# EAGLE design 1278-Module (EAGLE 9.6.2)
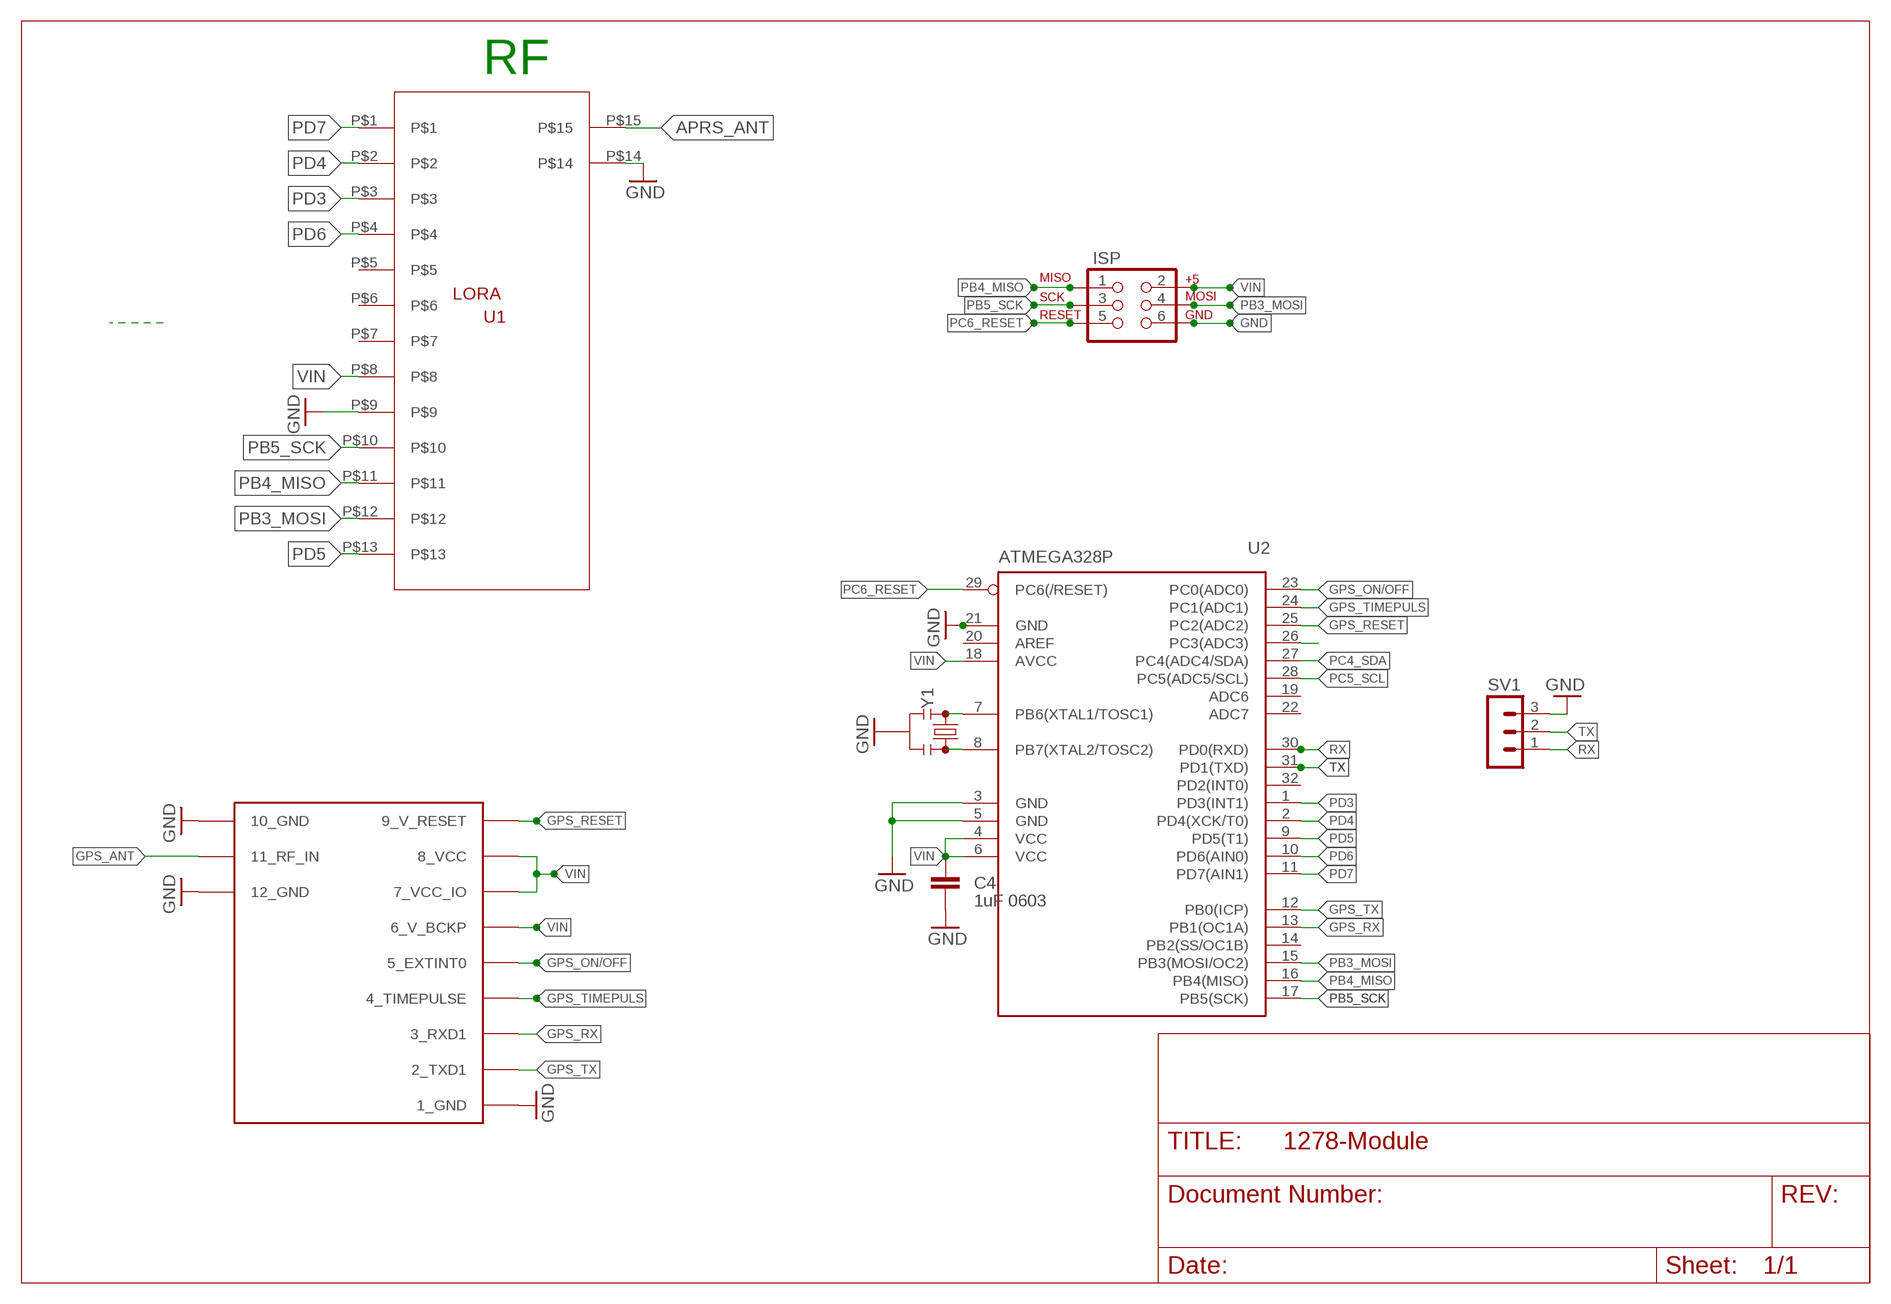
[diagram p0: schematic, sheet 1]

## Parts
C4  1uF 0603  C-EUC0603K  [C0603K]
ISP  AVR_SPI_PRG_6PTH  [2X3]
SV1  MA03-1  [MA03-1]
U1  LORA  [LORA_DRF]
U2  ATMEGA328P  MEGA8-AI  [TQFP32-08]
U$2  UBLOX_MAX  [UBLOX_MAX]
Y1  RESONATORSMD-4.5X2.0  [RESONATOR-SMD-4.5X2.0]

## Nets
APRS_ANT: U1.P$15
GND: C4.2 ISP.6 SV1.3 U1.P$9 U1.P$14 U2.3(GND) U2.5(GND) U2.21(GND) U$2.1_GND U$2.10_GND U$2.12_GND Y1.2
GPS_ANT: U$2.11_RF_IN
GPS_ON/OFF: U2.23(PC0(ADC0)) U$2.5_EXTINT0
GPS_RESET: U2.25(PC2(ADC2)) U$2.9_V_RESET
GPS_RX: U2.13(PB1(OC1A)) U$2.3_RXD1
GPS_TIMEPULS: U2.24(PC1(ADC1)) U$2.4_TIMEPULSE
GPS_TX: U2.12(PB0(ICP)) U$2.2_TXD1
N$1: U2.8(PB7(XTAL2/TOSC2)) Y1.3
N$2: U2.7(PB6(XTAL1/TOSC1)) Y1.1
N$10: U2.26(PC3(ADC3))
PB3_MOSI: ISP.4 U1.P$12 U2.15(PB3(MOSI/OC2))
PB4_MISO: ISP.1 U1.P$11 U2.16(PB4(MISO))
PB5_SCK: ISP.3 U1.P$10 U2.17(PB5(SCK))
PC4_SDA: U2.27(PC4(ADC4/SDA))
PC5_SCL: U2.28(PC5(ADC5/SCL))
PC6_RESET: ISP.5 U2.29(PC6(/RESET))
PD3: U1.P$3 U2.1(PD3(INT1))
PD4: U1.P$2 U2.2(PD4(XCK/T0))
PD5: U1.P$13 U2.9(PD5(T1))
PD6: U1.P$4 U2.10(PD6(AIN0))
PD7: U1.P$1 U2.11(PD7(AIN1))
RX: SV1.1 U2.30(PD0(RXD))
TX: SV1.2 U2.31(PD1(TXD))
VIN: C4.1 ISP.2 U1.P$8 U2.4(VCC) U2.6(VCC) U2.18(AVCC) U$2.6_V_BCKP U$2.7_VCC_IO U$2.8_VCC
Unconnected: U1.P$5 U1.P$6 U1.P$7 U2.14(PB2(SS/OC1B)) U2.19(ADC6) U2.20(AREF) U2.22(ADC7) U2.32(PD2(INT0))

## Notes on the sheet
- RF

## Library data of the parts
C4 = rcl:C-EU: CAPACITOR, European symbol; SPICEPREFIX: C
ISP = SparkFun:AVR_SPI_PRG_6: AVR ISP 6 Pin This is the reduced ISP connector for AVR programming. Common on Arduino. This footprint will take up less PCB space and can be used with a 10-pin to 6-pin adapter such as SKU: BOB-08508
SV1 = con-lstb:MA03-1: PIN HEADER; OC_FARNELL: unknown; OC_NEWARK: unknown
U1 = lora:LORA
U2 = atmel:MEGA8: MICROCONTROLLER 8 Kbytes FLASH, 1 kbytes SRAM, 512 bytes EEPROM, USART, 6-channel 10 bit ADC, 2-channel 8 bit ADC Pin compatible with Atmega48, ATMega88, ATMega168 Source: avr.lbr; MPN: ATMEGA8-16AU; OC_FARNELL: 9171371; OC_NEWARK: 73M8863
U$2 = Max gps:UBLOX_MAX: UBLOX MAX
Y1 = SparkFun-Clocks:RESONATOR: Resonators (Generic) Ceramic resonators are clock-generating components, often used to control timing in microcontrollers. They usually have 3 pins: two pins for oscillation, and one pin for ground. Compared to crystals, resonators have worse tolerance, but are usually much cheaper. Plus, they have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

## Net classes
0 default: width 0.152 mm, drill 0.305 mm, clearance 0.152 mm
1 vcc: width 0.152 mm, clearance 0.152 mm

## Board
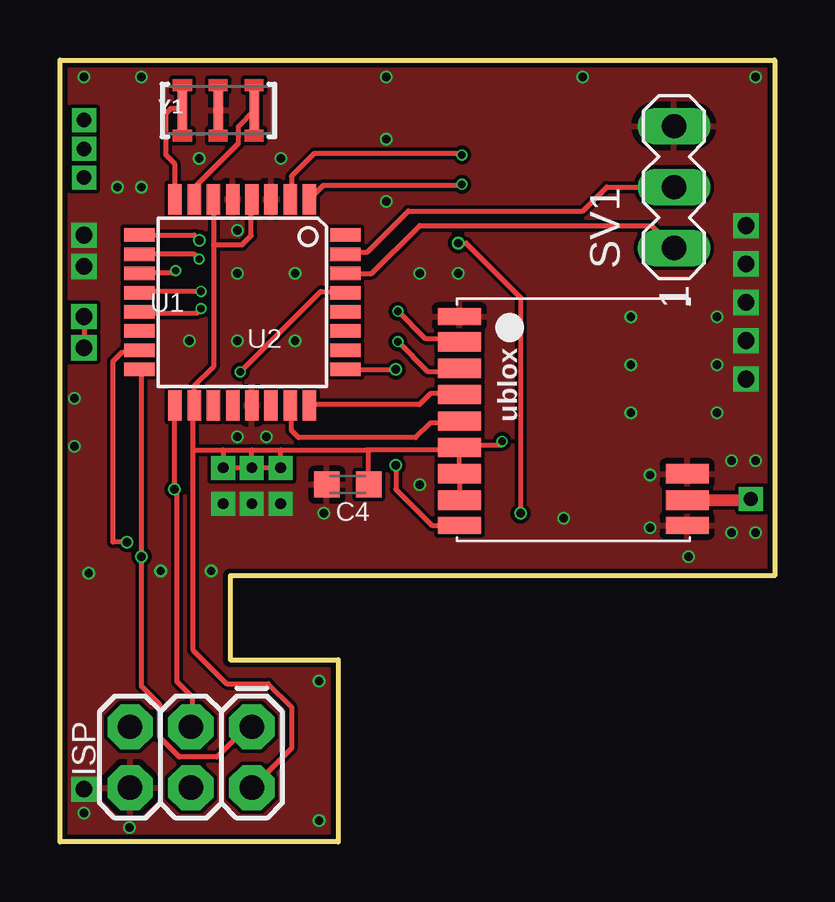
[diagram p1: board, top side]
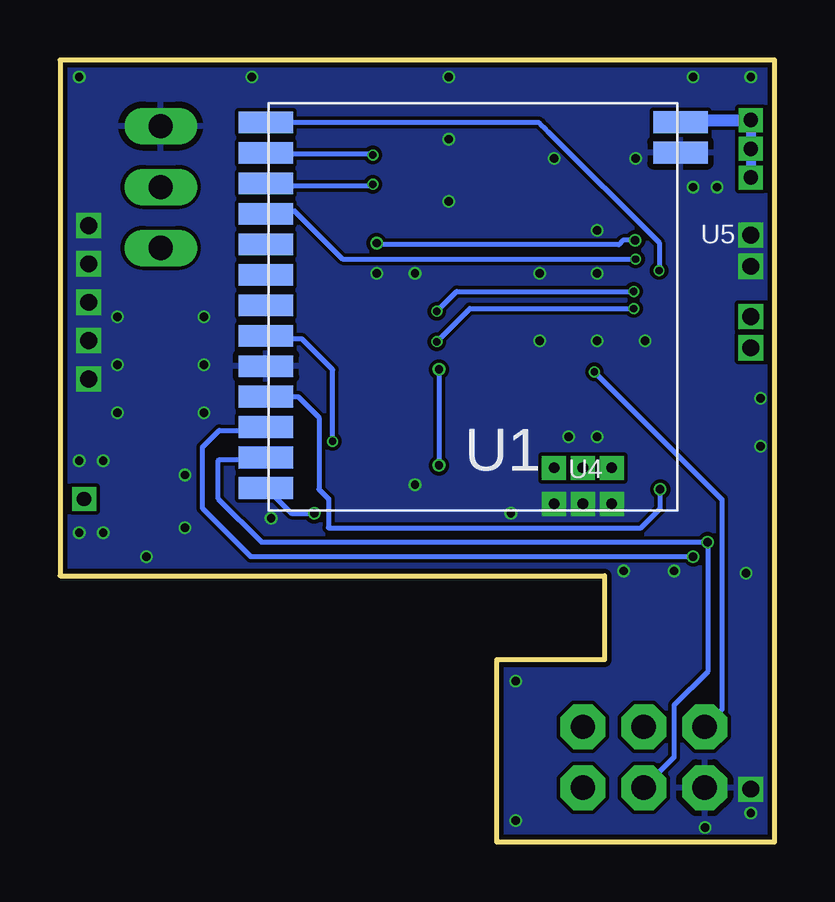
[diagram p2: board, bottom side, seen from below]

Size 29.8 x 32.6 mm. Coordinates in mm from the lower left corner, seen from the top.
Outline: 0,32.6 29.8,32.6 29.8,11.1 7.1,11.1 7.1,7.6 11.6,7.6 11.6,0 0,0 0,32.6
Copper layers (1*16): Top 0.035559375mm / dielectric 1.6mm / Bottom 0.035559375mm
Design rules "jlcpcb2layer *": minimum track width 5mil, minimum drill 12mil, track to track 5mil, track to pad 5mil, pad to pad 5mil, via to via 5mil, smd to smd 5mil, copper to edge 8mil, drill to drill 6mil, minimum pad ring 5mil, minimum via ring 3mil, stop-mask expansion 2.5mil, vias tented up to drill 14mil, thermal gap 10mil

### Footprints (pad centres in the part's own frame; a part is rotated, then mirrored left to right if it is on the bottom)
C0603K = smd 1.05 x 1.08: 1 -0.875,0; 2 0.875,0
2X3 = drill 1.016 pad 1.88 octagon: 1 0,0; 2 0,2.54; 3 2.54,0; 4 2.54,2.54; 5 5.08,0; 6 5.08,2.54
MA03-1 = drill 1.016 long: 1 -2.54,0; 2 0,0; 3 2.54,0
LORA_DRF = smd 2.27 x 0.9: P$1 -8.609,7.497; P$2 -8.609,6.227; P$3 -8.608,4.958; P$4 -8.608,3.688; P$5 -8.609,2.417; P$6 -8.609,1.147; P$7 -8.608,-0.122; P$8 -8.608,-1.392; P$9 -8.61,-2.663; P$10 -8.61,-3.933; P$11 -8.609,-5.202; P$12 -8.609,-6.472; P$13 -8.609,-7.743; P$14 8.673,6.235; P$15 8.675,7.506
TQFP32-08 = smd 1.27 x 0.559: 1 -4.293,2.8; 2 -4.293,2; 3 -4.293,1.2; 4 -4.293,0.4; 5 -4.293,-0.4; 6 -4.293,-1.2; 7 -4.293,-2; 8 -4.293,-2.8; 17 4.293,-2.8; 18 4.293,-2; 19 4.293,-1.2; 20 4.293,-0.4; 21 4.293,0.4; 22 4.293,1.2; 23 4.293,2; 24 4.293,2.8 | smd 0.559 x 1.27: 9 -2.8,-4.293; 10 -2,-4.293; 11 -1.2,-4.293; 12 -0.4,-4.293; 13 0.4,-4.293; 14 1.2,-4.293; 15 2,-4.293; 16 2.8,-4.293; 25 2.8,4.293; 26 2,4.293; 27 1.2,4.293; 28 0.4,4.293; 29 -0.4,4.293; 30 -1.2,4.293; 31 -2,4.293; 32 -2.8,4.293
UBLOX_MAX = smd 1.8 x 0.7: 1_GND 4.95,-4.4; 9_V_RESET 4.95,4.3; 10_GND -4.55,4.3 | smd 1.8 x 0.8: 2_TXD1 4.95,-3.35; 3_RXD1 4.95,-2.25; 4_TIMEPULSE 4.95,-1.15; 5_EXTINT0 4.95,-0.05; 6_V_BCKP 4.95,1.05; 7_VCC_IO 4.95,2.15; 8_VCC 4.95,3.25; 11_RF_IN -4.55,3.25; 12_GND -4.55,2.15
RESONATOR-SMD-4.5X2.0 = smd 0.4 x 1.6: 1 -1.5,0; 2 0,0; 3 1.5,0

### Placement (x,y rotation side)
C4  12,14.9 180 top
ISP  8,4.8 180 top
SV1  25.6,27.3 90 top
U1  12.6,22.5 0 bottom
U2  7.6,22.5 270 top
U$2  21.6,17.5 180 top
Y1  6.6,30.5 180 top

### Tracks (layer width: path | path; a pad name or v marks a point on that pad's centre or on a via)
APRS_ANT  (via drill 0.6 pad 1)
  Bottom 0.203: U1.P$15 3.83,30.1
  Bottom 0.406: v1,30.1 v1,28.9 v1,27.7
  Bottom 0.508: 3.83,30.1 v1,30.1
GND  (via drill 0.35, 0.45 pad 1, 0.7 pad 1)
  Top 0.203: U2.5 7.21,26.76 7.24,26.83
  other vias: 2.4,27.3 13.6,31.9 23.8,19.9 26.2,11.9 7.4,20.9 15,14.9 0.6,18.5 24.6,15.3 16.6,23.7 9.8,20.9 7.4,25.5 5.8,28.5 3.4,27.3 8.6,16.9 11,13.7 7.4,23.7 9.8,23.7 1,24 1,25.3 28.6,25.7 28.6,24.1 28.6,22.5 28.6,20.9 28.6,19.3 23.8,21.9 27.4,21.9 27.4,19.9 27.4,17.9 23.8,17.9 29,15.9 29,12.9 5.4,20.9 0.6,16.5 2.9,0.6 10.8,6.7 10.8,0.9 1,1.2 1.2,11.2 6.3,11.3 29,31.9 1,31.9 3.4,31.9 15,23.7 21.8,31.9 9.2,28.5 13.6,26.7 6.8,14.1 8,14.1 9.2,14.1 28,15.9 28,12.9 21,13.5 7.4,16.9 13.6,29.3 4.2,11.3 1,2.2 24.6,13.1
  pour Top: -4.79,41.22 49.15,41.22 49.15,-1.89 -4.79,-1.89
  pour Bottom: -4.79,41.22 49.15,41.22 49.15,-1.89 -4.79,-1.89
GPS_ANT  (via drill 0.6 pad 1)
  Top 0.203: 28.75,14.25 v28.8,14.3
  Top 0.508: U$2.11_RF_IN 28.75,14.25
GPS_ON/OFF
  Top 0.203: 16.51,17.46 16.54,17.46 16.64,17.56 | 16.51,17.46 15.44,17.46 14.83,16.86 9.96,16.86 9.65,17.16 9.65,18.07 9.62,18.21 9.65,18.23 U2.23 | 16.51,17.46 U$2.5_EXTINT0
GPS_RESET  (via drill 0.35)
  Top 0.203: U2.25 11.94,19.75 U2.25 v14,19.7 | v14,15.7 14,14.7 15.5,13.2 U$2.9_V_RESET
  Bottom 0.203: v14,19.7 v14,15.7
GPS_RX  (via drill 0.3)
  Top 0.203: v5.88,22.24 5.68,22.04 3.37,22.04 U2.13 3.4,22.04 3.39,22.04 U2.13 | v14.09,20.86 15.35,19.6 16.5,19.6 | 16.5,19.6 U$2.3_RXD1 | 16.5,19.6 16.51,19.6 U$2.3_RXD1
  Bottom 0.203: v5.88,22.24 12.71,22.24 v14.09,20.86
GPS_TIMEPULS
  Top 0.203: 16.51,18.68 15.44,18.68 14.98,18.23 10.42,18.23 10.41,18.23 | 10.41,18.23 U2.24 | 16.51,18.68 16.65,18.67 | U2.24 10.41,18.23 | 16.51,18.68 U$2.4_TIMEPULSE
GPS_TX  (via drill 0.3)
  Top 0.203: v5.88,22.95 3.4,22.95 | v14.09,22.12 15.24,20.97 16.51,20.97 | 16.51,20.97 16.52,20.97 U$2.2_TXD1 | 3.32,22.89 3.38,22.95 3.4,22.95 | 3.4,22.95 U2.12 | 16.51,20.97 U$2.2_TXD1
  Bottom 0.203: v5.88,22.95 13.26,22.95 v14.09,22.12
N$1
  Top 0.203: 5.08,30.57 5.09,30.57 Y1.3 | 5.08,30.57 4.62,30.57 4.41,30.36 4.41,28.65 4.77,28.29 4.77,26.91 4.79,26.79 4.77,26.76 U2.8 | 5.08,30.57 Y1.3
N$2
  Top 0.203: Y1.1 7.43,29.83 7.43,29.11 5.54,27.21 5.54,26.89 5.61,26.81 U2.7
N$7  (via drill 0.7 pad 1)
  Top 0.203: v1,21.9 v1,20.6
PB3_MOSI  (via drill 0.35)
  Top 0.203: U2.15 3.25,20.51 3.29,20.51 U2.15 3.21,20.41 2.58,20.41 2.2,20.03 2.2,12.5 v2.8,12.5
  Bottom 0.203: U1.P$12 21.23,15.94 23.16,15.94 23.2,15.9 23.2,14.3 21.4,12.5 v2.8,12.5 2.8,7.1 4.2,5.7 4.2,3.52 ISP.4
PB4_MISO  (via drill 0.35)
  Top 0.203: v3.4,11.9 3.4,6.49 4.16,5.73 4.16,4.36 4.98,3.54 6.55,3.54 7.67,4.66 7.97,4.66 ISP.1 | v3.4,11.9 3.4,19.6 | 3.4,19.6 U2.16 | 3.4,19.6 U2.16 | v3.4,11.9
  Bottom 0.203: U1.P$11 21.21,17.16 23.16,17.16 23.86,16.45 23.86,13.91 21.85,11.9 v3.4,11.9
PB5_SCK  (via drill 0.35)
  Top 0.203: ISP.3 5.54,4.82 5.54,6.03 4.87,6.7 4.87,14.6 v4.77,14.7 4.77,18.07 4.79,18.21 4.77,18.23 U2.17
  Bottom 0.203: v4.77,14.7 4.77,13.9 5.57,13.1 18.6,13.1 18.6,14.3 19,14.7 19,17.7 19.87,18.57 U1.P$10
PC6_RESET  (via drill 0.3)
  Top 0.203: 11.78,22.95 10.87,22.95 v7.52,19.6 | 11.78,22.95 11.81,22.95 11.88,22.89 | 11.78,22.95 U2.29
  Bottom 0.203: ISP.5 2.2,5.52 2.2,14.28 v7.52,19.6
PD3  (via drill 0.3)
  Top 0.203: v16.76,27.42 16.7,27.36 10.97,27.36 U2.1 10.41,26.76 U2.1
  Bottom 0.203: v16.76,27.42 16.8,27.37 21.08,27.37 U1.P$3
PD4  (via drill 0.3)
  Top 0.203: 9.65,26.91 9.65,27.75 10.6,28.7 16.69,28.7 v16.76,28.64 | 9.58,26.81 9.65,26.88 9.65,26.91 | 9.65,26.91 U2.2
  Bottom 0.203: v16.76,28.64 16.82,28.7 21.18,28.7 U1.P$2
PD5  (via drill 0.35)
  Top 0.203: v19.2,13.7 19.2,22.7 16.93,24.97 v16.6,24.97 | U2.9 5.6,25.3 v5.82,25.08
  Bottom 0.203: U1.P$13 20.15,13.7 v19.2,13.7 | v5.82,25.08 6.32,25.08 6.5,24.9 16.53,24.9 v16.6,24.97
PD6  (via drill 0.3)
  Top 0.203: 3.31,24.49 3.4,24.48 U2.10 5.6,24.5 v5.8,24.3
  Bottom 0.203: v5.8,24.3 18.01,24.3 20.01,26.3 21.08,26.3 U1.P$4
PD7  (via drill 0.3)
  Top 0.203: 3.4,23.71 4.72,23.71 v4.82,23.82 | 3.4,23.71 U2.11 | 3.4,23.71 U2.11
  Bottom 0.203: v4.82,23.82 4.82,24.98 9.47,29.63 9.57,29.73 9.77,29.93 9.84,30 U1.P$1 21.08,29.96 20.93,29.81
RX
  Top 0.203: U2.30 13,23.7 15,25.7 24.66,25.7 SV1.1
TX
  Top 0.203: U2.31 11.99,24.59 12.82,24.59 14.53,26.3 21.8,26.3 22.8,27.3 SV1.2
VIN  (via drill 0.3, 0.45 pad 1)
  Top 0.203: 16.66,15.33 16.66,15.34 U$2.7_VCC_IO | 16.66,15.33 16.66,14.26 | U$2.8_VCC 16.66,14.26 | v18.43,16.7 18.43,16.55 16.66,16.55 | 16.66,16.55 U$2.6_V_BCKP 16.66,16.4 16.66,15.48 U$2.7_VCC_IO 16.66,15.33 | 7.97,26.91 7.97,26.9 | 7.97,26.9 7.99,26.79 | 6.4,24.9 U2.6 6.45,26.76 6.45,26.75 U2.6 | 6.4,24.9 6.4,19.81 5.6,19.01 U2.18 | U2.18 5.54,18.22 5.54,18.23 U2.18 | 7.97,26.76 U2.4 | 5.54,16.35 5.54,18.11 5.62,18.19 5.69,18.23 U2.18 | 5.54,16.35 5.54,8.02 6.95,6.6 8.68,6.6 9.65,5.62 9.65,3.9 8.13,2.38 ISP.2 | 5.54,16.35 6.8,16.35 | 6.8,16.35 8,16.35 | 8,16.35 9.2,16.35 | 9.2,16.35 12.8,16.35 | U$2.6_V_BCKP 16.55,16.35 12.8,16.35 | U$2.6_V_BCKP 16.53,16.55 16.51,16.55 U$2.6_V_BCKP | 16.66,14.26 U$2.8_VCC | 16.66,15.33 U$2.7_VCC_IO | 16.66,16.55 U$2.6_V_BCKP | 7.97,26.76 U2.4 7.97,26.82 7.97,26.9 | 6.4,24.9 7.6,24.9 7.97,25.27 7.97,26.76 | C4.1 12.87,16.27 12.8,16.35 | 6.8,16.35 v6.8,15.6 v8,15.6 | v8,15.6 v9.2,15.6 9.2,16.35 | v8,15.6 8,16.35
  Bottom 0.203: v18.43,16.7 18.43,19.69 19.71,20.97 21.08,20.97 U1.P$8

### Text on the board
tNames: U1
bNames: U5 | U4

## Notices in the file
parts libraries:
SparkFun-Clocks: Licensing: Creative Commons ShareAlike 4.0 International - https://creativecommons.org/licenses/by-sa/4.0
